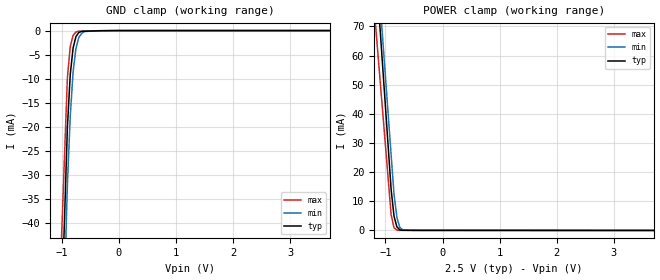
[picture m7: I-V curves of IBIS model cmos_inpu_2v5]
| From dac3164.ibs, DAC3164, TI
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[Model] cmos_inpu_2v5
Model_type Input
Vinl = 750.000mV
Vinh = 1.50000V
C_comp 865.000fF 865.000fF 865.000fF
| variable typ   min   max
[Voltage Range] 2.50000V 2.25000V 2.75000V
[POWER Clamp Reference] 2.50000V 2.25000V 2.75000V
[GND Clamp Reference] 0.00000V 0.00000V 0.00000V
[Temperature Range]   25   85   -40
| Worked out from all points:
|   GND clamp passes 1 mA (typ) near -0.74 V on its own axis
|   POWER clamp passes 1 mA (typ) near -0.79 V on its own axis
[GND Clamp]
-2.5V     -624.1mA   -694.2mA   -528.4mA
-900mV    -20.08mA   -32mA      -9.755mA
-850mV    -9.125mA   -17.77mA   -3.35mA
-800mV    -3.595mA   -8.557mA   -996.6uA
-750mV    -1.243mA   -3.658mA   -297uA
-700mV    -401.1uA   -1.439mA   -130.9uA
-650mV    -154uA     -567.7uA   -115.8uA
-600mV    -135.3uA   -190.4uA   -100.6uA
0V        0A         0A         0A
5V        0A         0A         0A
[POWER Clamp]
-2.5V     469.7mA    456.5mA    387.7mA
-1.15V    85.16mA    93.14mA    65.01mA
-1.1V     70.92mA    79.68mA    53.05mA
-1.05V    56.68mA    66.22mA    41.1mA
-900mV    13.95mA    25.85mA    5.246mA
-850mV    4.911mA    12.4mA     908.6uA
-800mV    1.231mA    4.497mA    112.6uA
-750mV    197.9uA    1.07mA     13.73uA
-700mV    29.31uA    208.1uA    12.36uA
-600mV    20.94uA    26.8uA     9.611uA
5V        -36.22uA   -36.56uA   -30.94uA
